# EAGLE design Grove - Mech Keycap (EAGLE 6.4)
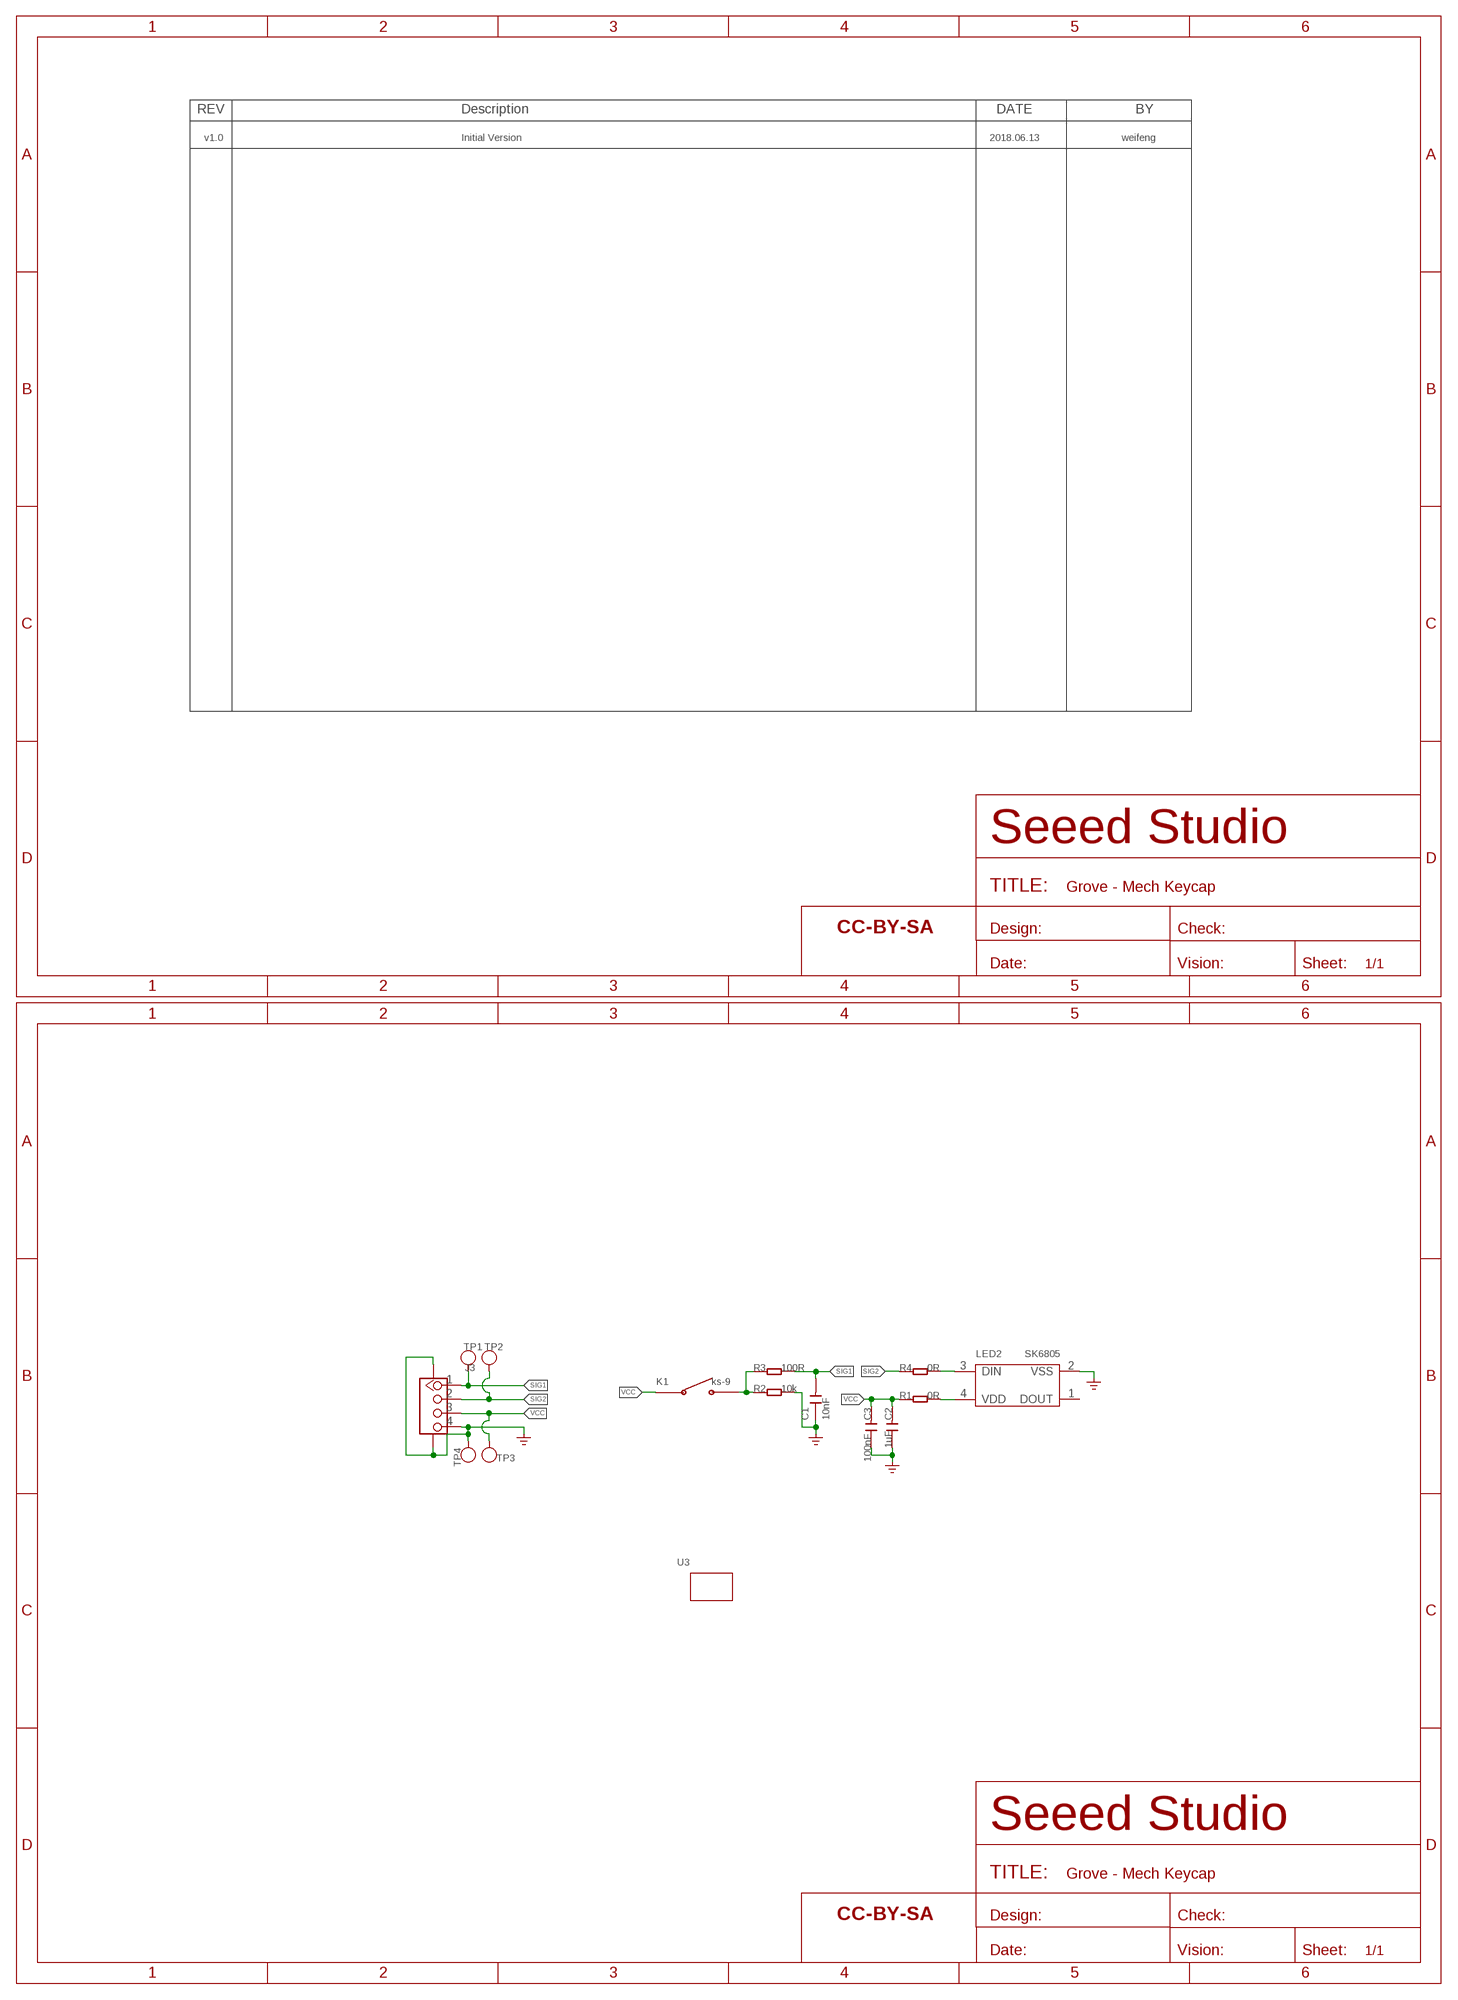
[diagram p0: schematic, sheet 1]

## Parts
C1  10nF  CAP-0603  [C0603]
C2  1uF  CAP-0603  [C0603]
C3  100nF  CAP-0603  [C0603]
FR1  SEEEDSTUDIO-OPEN-SCH-FRAME  [SEEEDSTUDIO-PCB-FRAME]
J3  GROVE-CONNECTOR-SMD'DD'  [HW4-SMD-2.0]
K1  ks-9  BUTTON-KS-9'3.9'  [LOW1]
LED2  SK6805  LED-SK6805-2427  [LED-4P-SMD-2.7X2.4MM]
R1  0R  RES-0603  [R0603]
R2  10k  RES-0603  [R0603]
R3  100R  RES-0603  [R0603]
R4  0R  RES-0603  [R0603]
TP1  TEST-POINT'4545'  [TP-D45MIL]
TP2  TEST-POINT'4545'  [TP-D45MIL]
TP3  TEST-POINT'4545'  [TP-D45MIL]
TP4  TEST-POINT'4545'  [TP-D45MIL]
U3  GROVE-1X1-TOP  [GROVE-1X1-TEST-PLATFORM-TOP]
U$4  SEEEDSTUDIO-OPEN-SCH-FRAME  [SEEEDSTUDIO-PCB-FRAME]

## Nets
GND: C1.1 C2.1 C3.1 J3.4 J3.SS1 J3.SS2 LED2.2(VSS) R2.2 TP4.T ; supply symbol labelled GND_POWER
N$1: LED2.4(VDD) R1.2
N$2: K1.2 R2.1 R3.1
N$3: LED2.3(DIN) R4.2
SIG1: C1.2 J3.1 R3.2 TP1.T
SIG2: J3.2 R4.1 TP2.T
VCC: C2.2 C3.2 J3.3 K1.1 R1.1 TP3.T
Unconnected: LED2.1(DOUT)

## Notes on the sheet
- v1.0 | Initial Version | 2018.06.13 | weifeng

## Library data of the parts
C1-C3 = Discrete-new:CAP: Ceramic Capacitors
FR1 U$4 = moudle-new:SEEEDSTUDIO-OPEN-SCH-FRAME
J3 = Connector-new:GROVE-CONNECTOR-SMD: 4P-SMD-2.0:320110030;4P-SMD-2.0-90D:320110032
K1 = Discrete-new:BUTTON-KS-9
LED2 = template:LED-SK6805-2427
R1-R4 = Discrete-new:RES
TP1-TP4 = Discrete-new:TEST-POINT; PARTNO: DNP
U3 = moudle-new:GROVE

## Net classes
3 usbvcc: width 0.203 mm, drill 0.305 mm, clearance 0.203 mm

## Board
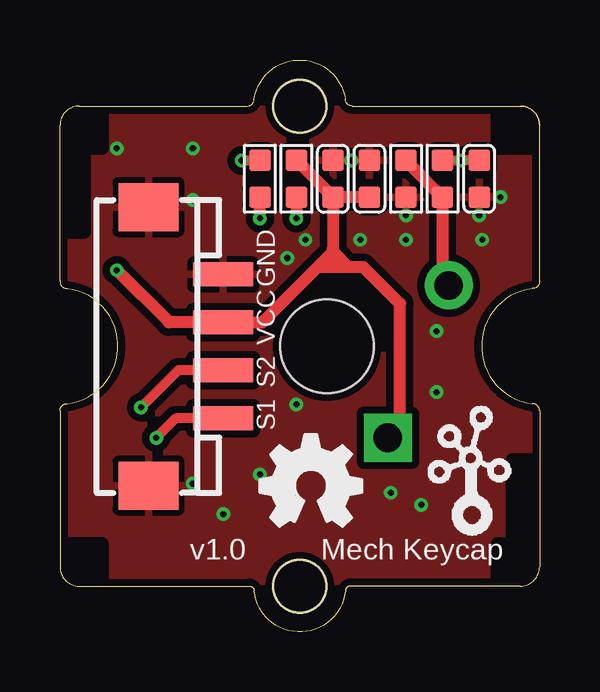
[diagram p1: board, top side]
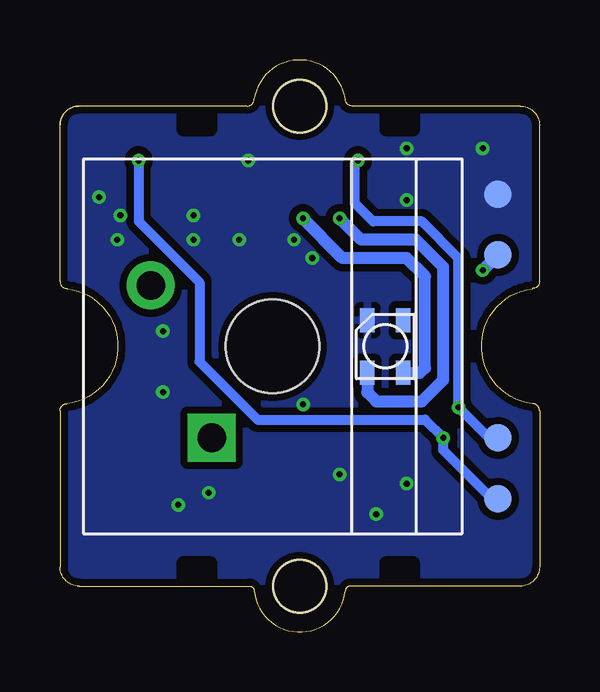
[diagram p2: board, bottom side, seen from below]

Size 20 x 23.83 mm. Coordinates in mm from the lower left corner, seen from the top.
Copper layers (1*16): Top 0.035mm / dielectric 1.5mm / Bottom 0.035mm
Design rules "SeeedStudio_2layer_DRU_no_angle_20140221 *": minimum track width 6mil, minimum drill 10mil, track to track 6mil, track to pad 6mil, pad to pad 6mil, via to via 6mil, smd to smd 0mil, copper to edge 10mil, drill to drill 10mil, minimum pad ring 10mil, minimum via ring 6mil, stop-mask expansion 2mil, vias tented up to drill 25mil, thermal gap 10mil

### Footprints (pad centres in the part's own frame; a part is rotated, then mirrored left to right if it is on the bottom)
C0603 = smd 0.889 x 0.889: 1 0,0.762; 2 0,-0.762
HW4-SMD-2.0 = smd 1 x 2.5: 1 -3,0; 2 -1,0; 3 1,0; 4 3,0 | smd 2 x 2.5: SS1 -5.8,3.123; SS2 5.8,3.123
LOW1 = drill 1.2 pad 2 square: 1 -3.81,2.54 | drill 1.2 pad 2: 2 2.54,5.08 | hole 3.9: 0,0
LED-4P-SMD-2.7X2.4MM = smd 1 x 0.6: 1 1.1,-0.75; 2 1.1,0.75; 3 -1.1,0.75; 4 -1.1,-0.75
R0603 = smd 0.889 x 0.889: 1 0,0.762; 2 0,-0.762
TP-D45MIL = smd 1.143 x 1.143: T 0,0
GROVE-1X1-TEST-PLATFORM-TOP = hole 2.2: 9.987,0.013; -10.013,0.013

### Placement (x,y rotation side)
C1  17.48,18.88 180 top
C2  12.91,18.88 0 top
C3  11.38,18.88 0 top
FR1  not placed on the board
J3  6.81,11.9 90 top
K1  11.13,11.9 90 bottom
LED2  6.43,11.9 90 bottom
R1  9.86,18.88 0 top
R2  14.43,18.88 0 top
R3  15.96,18.88 180 top
R4  8.34,18.88 0 top
TP1  1.73,5.55 0 bottom
TP2  1.73,8.09 0 bottom
TP3  1.73,15.71 0 bottom
TP4  1.73,18.25 0 bottom
U3  9.99,11.9 270 top
U$4  not placed on the board
U$9  [OSHW_FILLX150_NOTEXT]  8.34,4.4 0 top
U$10  [GROVE-SILK-SMALL]  14.94,3.89 0 top

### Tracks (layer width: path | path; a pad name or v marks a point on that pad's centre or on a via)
GND  (via drill 0.25 pad 0.51)
  other vias: 10.24,16.34 12.15,19.64 14.43,17.36 17.48,17.36 5.54,17.99 9.48,15.58 5.54,6.18 5.54,20.15 2.37,20.15 12.53,16.34 14.43,16.34 17.61,16.34 15.7,12.53 15.7,9.99 15.07,5.29 6.81,4.91 9.86,9.48 8.34,6.56 13.8,5.8 18.37,18.12
  pour Top (isolate 0.305): -1.44,23.96 20.15,23.71 20.15,-0.17 -1.44,-0.42
  pour Bottom (isolate 0.305): -1.44,23.96 20.15,23.71 20.15,-0.17 -1.44,-0.42
N$1  (via drill 0.25 pad 0.51)
  Top 0.508: R1.2 v9.86,17.23
  Bottom 0.508: LED2.4 4.99,10.8 4.78,11.01 4.78,14.82 5.54,15.58 8.21,15.58 v9.86,17.23
N$2
  Top 0.508: K1.2 15.96,14.69 R3.1 R2.1
N$3  (via drill 0.25 pad 0.51)
  Top 0.508: v8.34,17.23 R4.2
  Bottom 0.508: LED2.3 7.18,9.98 6.81,9.61 4.91,9.61 4.02,10.5 4.02,15.2 5.16,16.34 7.45,16.34 v8.34,17.23
SIG1  (via drill 0.25 pad 0.51)
  Top 0.406: J3.1 4.83,8.9 v4.02,8.09 | C1.2 v16.72,19.64 R3.2
  Bottom 0.406: TP1.T 1.99,5.55 4.02,7.58 v4.02,8.09 4.78,8.85 11.77,8.85 14.18,11.26 14.18,14.56 16.72,17.1 v16.72,19.64
SIG2  (via drill 0.25 pad 0.51)
  Top 0.406: J3.2 4.92,10.9 v3.38,9.36 | v7.57,19.64 R4.1
  Bottom 0.406: v7.57,19.64 7.7,19.52 7.7,17.86 6.94,17.1 4.91,17.1 3.38,15.58 v3.38,9.36 2.11,8.09 TP2.T
VCC  (via drill 0.25 pad 0.51)
  Top 0.508: 10.75,15.2 8.45,12.9 J3.3 4.54,12.9 v2.37,15.07 | C3.2 11.38,15.96 11.38,15.83 | 11.38,15.83 11.38,15.2 | C2.2 C3.2 | R1.1 C3.2 | K1.1 14.18,8.59 14.18,13.67 12.65,15.2 12.02,15.2 | 12.02,15.2 11.38,15.2 | 11.38,15.2 10.75,15.2 | 11.38,15.83 10.75,15.2 | 11.38,15.83 12.02,15.2
  Bottom 0.508: v2.37,15.07 TP3.T

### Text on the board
tPlace: GND | VCC | S2 | S1 | v1.0 | Mech Keycap

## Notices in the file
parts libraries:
moudle-new: This work is licensed under the Creative Commons Attribution 4.0 International License.
To view a copy of this license,visit:
http://creativecommons.org/licenses/by-sa/4.0
moudle-new: CC-BY-SA
